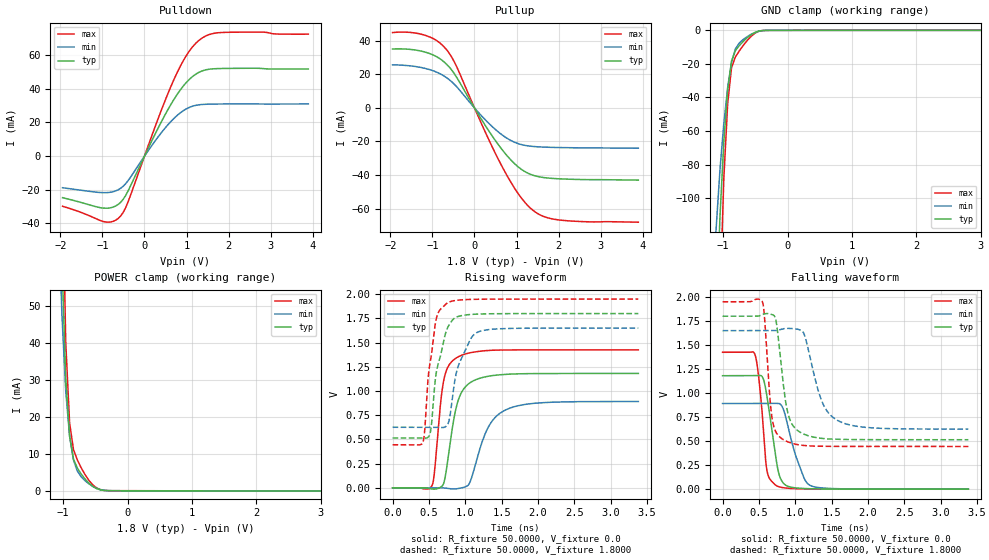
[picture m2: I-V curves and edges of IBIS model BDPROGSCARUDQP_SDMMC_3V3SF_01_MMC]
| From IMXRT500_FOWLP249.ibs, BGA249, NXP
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[Model] BDPROGSCARUDQP_SDMMC_3V3SF_01_MMC
|   Model BDPROGSCARUDQP_SDMMC_3V3SF_01_MMC
| This model was characterised for following simulation conditions:
| External (pad) voltage:
|   - Typ: 1.8V,   - Min: 1.65V,   - Max: 1.95V
| Library cells for typ/min/max conditions are connected as defined below:
|  IO - External Pad
|  A - Core Input
|  EN - Output Buffer Enable
|  ASRCN3V3[0] - REFH3V3
|  ASRCN3V3[1] - REFH3V3
|  ASRCN3V3[2] - REFH3V3
|  ASRCN3V3[3] - REFH3V3
|  ASRCP3V3[0] - REFL3V3
|  ASRCP3V3[1] - REFL3V3
|  ASRCP3V3[2] - REFL3V3
|  ASRCP3V3[3] - REFL3V3
|  IOGC - NC
|  PDRV - vdd
|  PSW - gnd
|  REFH3V3 - REFH3V3
|  REFL3V3 - REFL3V3
|  ZI - NC
|  gnd - gnd
|  gnde - gnde
|  vdd - vdd
|  vdde3v3 - vdde3v3
| All other pins connected to ground
Model_type I/O
Polarity   Non-Inverting
Enable   Active-Low
Vinl =   0.5775V
Vinh =   1.2675V
Vmeas =  0.9000V
Cref =   30.0000pF
Rref =   1.0000M
Vref =   1.8000V
C_comp   2.2202pF   2.2061pF   2.2431pF
|C_comp_pullup   1.1645pF   1.1333pF   1.1987pF
|C_comp_pulldown   0.0F   0.0F   0.0F
[Model Spec]
| variable   typ   min   max
Vinh   1.1700V   1.0725V   1.2675V
Vinl   0.6300V   0.5775V   0.6825V
|[Receiver Thresholds]
[Temperature Range]   25.0000   0.1050k   -20.0000
[Voltage Range]   1.8000V   1.6500V   1.9500V
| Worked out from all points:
|   slope of the pulldown table from 0 to 0.27 V, typ, clamps not added: 19.4 ohm
|   slope of the pullup table from 0 to 0.27 V, typ, clamps not added: 24.6 ohm
|   GND clamp passes 1 mA (typ) near -0.49 V on its own axis
|   POWER clamp passes 1 mA (typ) near -0.52 V on its own axis
|   rising waveform, R_fixture 50.0000, V_fixture 0.0: 20-80 % time 173ps typ, 278ps min, 121ps max; typ from 0 V to 1.18 V
|   rising waveform, R_fixture 50.0000, V_fixture 1.8000: 20-80 % time 161ps typ, 209ps min, 123ps max; typ from 0.514 V to 1.8 V
|   falling waveform, R_fixture 50.0000, V_fixture 0.0: 20-80 % time 137ps typ, 208ps min, 93.4ps max; typ from 1.18 V to 0 V
|   falling waveform, R_fixture 50.0000, V_fixture 1.8000: 20-80 % time 134ps typ, 241ps min, 89.4ps max; typ from 1.8 V to 0.514 V
[Pulldown]
|Voltage   I(typ)   I(min)   I(max)
-1.95V    -24.68mA   -18.78mA   -29.78mA
-930mV    -30.94mA   -21.7mA    -39.1mA
-750mV    -30.29mA   -21.15mA   -38.76mA
-570mV    -27.47mA   -19.13mA   -35.64mA
-390mV    -20.65mA   -14.54mA   -27.12mA
330mV     16.93mA    11.62mA    22.64mA
690mV     33.26mA    22.15mA    44.91mA
1.05V     45.2mA     28.77mA    61.79mA
1.35V     50.41mA    30.65mA    69.81mA
1.59V     51.79mA    30.91mA    72.62mA
1.89V     52.1mA     31mA       73.52mA
3.9V      51.78mA    31.01mA    72.47mA
[Pullup]
|Voltage   I(typ)   I(min)   I(max)
-1.95V    35.12mA    25.68mA    44.93mA
-1.2V     33.44mA    23.71mA    43.46mA
-900mV    30.51mA    21.31mA    40.14mA
-660mV    25.95mA    17.94mA    34.55mA
-420mV    18.07mA    12.52mA    24.35mA
180mV     -7.408mA   -5.025mA   -10.16mA
660mV     -24.94mA   -16.13mA   -35.07mA
1.02V     -34.7mA    -21.11mA   -50.34mA
1.38V     -40mA      -22.93mA   -60.76mA
1.68V     -41.59mA   -23.38mA   -64.99mA
2.04V     -42.27mA   -23.61mA   -66.84mA
3.9V      -43.01mA   -24.02mA   -68.09mA
[GND_clamp]
|Voltage   I(typ)   I(min)   I(max)
-1.95V    -1.765A    -1.022A    -2.885A
-1.11V    -175mA     -118.7mA   -274.2mA
-1.05V    -111.7mA   -83.43mA   -161.8mA
-990mV    -66.62mA   -55.67mA   -88.75mA
-930mV    -35.53mA   -34.14mA   -43.79mA
-870mV    -18.33mA   -19.05mA   -22.29mA
-810mV    -12.12mA   -11.08mA   -15.87mA
-750mV    -9.12mA    -7.575mA   -12.28mA
-570mV    -2.717mA   -2.477mA   -3.751mA
-450mV    -466.5uA   -625uA     -610.9uA
-330mV    -31.46uA   -57.07uA   -36.76uA
3.9V      0A         0A         0A
[POWER_clamp]
|Voltage   I(typ)   I(min)   I(max)
-1.95V    1.71A      976mA      2.836A
-1.08V    122.1mA    81.01mA    201.9mA
-1.02V    63.03mA    48mA       94.76mA
-960mV    30.4mA     27.02mA    40.25mA
-900mV    14.88mA    14.82mA    18.42mA
-840mV    8.668mA    8.369mA    11.21mA
-780mV    6.192mA    5.372mA    8.379mA
-720mV    4.573mA    3.84mA     6.25mA
-600mV    2.107mA    1.918mA    2.859mA
-480mV    625.6uA    714.7uA    800.1uA
-300mV    67.29uA    79.42uA    85.49uA
3.9V      0A         0A         0A
[Ramp]
| variable   typ   min   max
dV/dt_r  0.7082/0.1727n   0.5346/0.2785n   0.8544/0.1206n
dV/dt_f  0.7708/0.1340n   0.6145/0.2411n   0.9029/89.3861p
R_load = 50.0000
[Rising Waveform]
R_fixture= 50.0000
V_fixture= 0.0
V_fixture_min= 0.0
V_fixture_max= 0.0
|time   V(typ)   V(min)   V(max)
0s        140.6uV    132.3uV    166.9uV
541.6ps   -12.52mV   112uV      21.29mV
574.2ps   -14.31mV   158.4uV    147.6mV
659.2ps   6.145mV    515.2uV    864.5mV
703.8ps   47.32mV    -1.349mV   1.11V
887.9ps   865.7mV    -9.576mV   1.347V
1.051ns   1.077V     38.87mV    1.392V
1.296ns   1.149V     596.1mV    1.417V
1.55ns    1.171V     802.6mV    1.423V
3.38ns    1.18V      891.1mV    1.424V
[Rising Waveform]
R_fixture= 50.0000
V_fixture= 1.8000
V_fixture_min= 1.6500
V_fixture_max= 1.9500
|time   V(typ)   V(min)   V(max)
0s        514.5mV    625mV      444.3mV
417.7ps   514.5mV    625.1mV    470mV
440.7ps   513.6mV    625.1mV    579.6mV
489.7ps   522.3mV    625.1mV    1.14V
522.3ps   581.3mV    625.2mV    1.318V
593.7ps   1.151V     625.3mV    1.72V
762.7ps   1.662V     662.3mV    1.914V
892.5ps   1.767V     1.231V     1.937V
1.153ns   1.794V     1.601V     1.947V
3.38ns    1.799V     1.649V     1.949V
[Falling Waveform]
R_fixture= 50.0000
V_fixture= 0.0
V_fixture_min= 0.0
V_fixture_max= 0.0
|time   V(typ)   V(min)   V(max)
0s        1.18V      891.2mV    1.424V
444.6ps   1.18V      891.3mV    1.403V
510.1ps   1.182V     891.4mV    1.074V
560.2ps   1.148V     891.3mV    633.9mV
605.9ps   987.5mV    891.1mV    213.6mV
742.3ps   283.6mV    892.6mV    36.14mV
863.5ps   43.76mV    763.8mV    12.5mV
1.025ns   12.07mV    308mV      4.788mV
1.217ns   4.434mV    34.57mV    1.841mV
3.38ns    145.1uV    222.3uV    167.7uV
[Falling Waveform]
R_fixture= 50.0000
V_fixture= 1.8000
V_fixture_min= 1.6500
V_fixture_max= 1.9500
|time   V(typ)   V(min)   V(max)
0s        1.799V     1.649V     1.949V
549.2ps   1.818V     1.649V     1.948V
678.8ps   1.817V     1.649V     748.5mV
741.4ps   1.725V     1.651V     584.1mV
835.2ps   1.094V     1.669V     515.3mV
1.001ns   630.7mV    1.668V     468.4mV
1.124ns   570.6mV    1.608V     453.4mV
1.385ns   526.8mV    880.2mV    446mV
1.577ns   518.8mV    716.8mV    444.8mV
3.38ns    514.5mV    625mV      444.3mV
